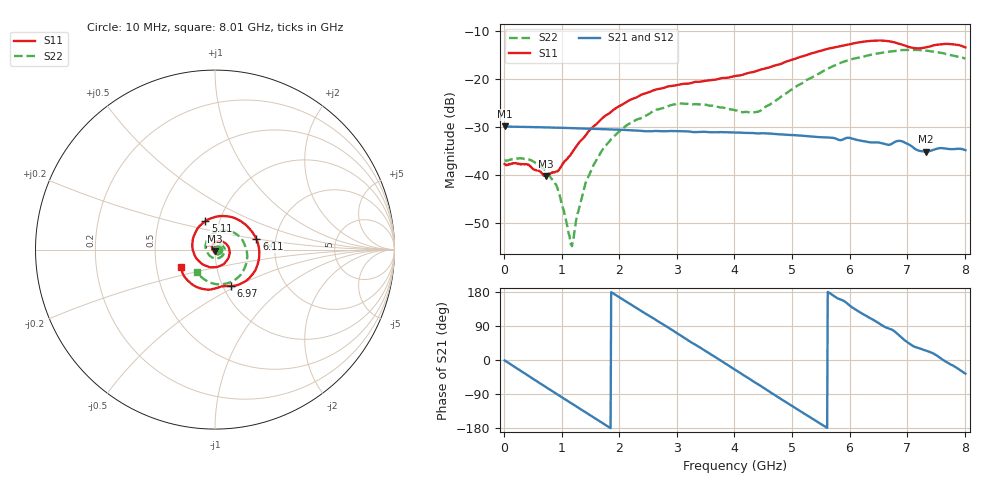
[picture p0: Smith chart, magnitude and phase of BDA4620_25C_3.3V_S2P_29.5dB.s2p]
!Agilent Technologies,E5071B,MY42404982,A.09.10
!Date: Wed May 06 08:55:15 2026
!Data & Calibration Information:
!Freq	S11:SOLT2(ON)	S21:SOLT2(ON)	S12:SOLT2(ON)	S22:SOLT2(ON)
# Hz S RI R 50
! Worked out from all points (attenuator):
!   801 points, 10 MHz to 8.01 GHz, reference 50 ohm
!   highest |S21| = -29.86 dB at 10 MHz (marker M1); lowest = -35.1 dB at 7.33 GHz (marker M2)
!   lowest |S11| = -40.2 dB at 720 MHz (marker M3), VSWR 1.02, Z = 49.8 - j0.961 ohm
!   |S11| at or under -10 dB: start of sweep to end of sweep
!   |S22| runs from -54.8 to -13.9 dB; largest |S21 - S12| = 0.0002
!   S11 on the Smith chart (normalised r, x): 10 MHz: 1.03, -0.00; 5.11 GHz: 0.86, +0.28; 6.11 GHz: 1.59, +0.19; 6.97 GHz: 1.09, -0.47; 8.01 GHz: 0.67, -0.14
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1e7  0.013 -0.000746  0.0321 -0.000672  0.0322 -0.000656  0.014 -0.000464
4.4e8  0.00856 -0.00926  0.023 -0.0218  0.023 -0.0218  0.0135 -0.00514
7.2e8  -0.00148 -0.00964  0.0103 -0.0296  0.0103 -0.0296  0.00851 -0.00729
9.3e8  -0.00959 -0.00526  -0.000679 -0.0311  -0.000697 -0.0311  0.00356 -0.00631
1.17e9  -0.0157 0.00595  -0.0128 -0.0281  -0.0129 -0.0281  -0.00158 -0.00111
1.2e9  -0.0161 0.00773  -0.0142 -0.0273  -0.0142 -0.0273  -0.00206 -8.8e-05
1.35e9  -0.0163 0.0168  -0.0204 -0.0228  -0.0204 -0.0228  -0.00355 0.00452
1.53e9  -0.0119 0.0288  -0.026 -0.0155  -0.0261 -0.0155  -0.00347 0.0112
1.77e9  0.00163 0.0418  -0.0297 -0.00404  -0.0298 -0.00404  0.000624 0.0204
2.15e9  0.0364 0.0462  -0.0258 0.0142  -0.0258 0.0143  0.0169 0.0292
2.68e9  0.0786 0.00593  -0.00575 0.0281  -0.00574 0.0282  0.0442 0.0196
3.08e9  0.0736 -0.0494  0.0128 0.0255  0.0129 0.0256  0.0551 -0.00704
4.01e9  -0.071 -0.0807  0.025 -0.012  0.0251 -0.0121  -0.0101 -0.0464
4.43e9  -0.1239 -0.00181  0.0111 -0.0248  0.0111 -0.0249  -0.0447 -0.0118
5.11e9  -0.054 0.1587  -0.0172 -0.0193  -0.0173 -0.0193  -0.0168 0.0848
5.35e9  0.0162 0.1852  -0.0228 -0.0107  -0.0228 -0.0107  0.0228 0.1016
6.11e9  0.2311 0.0574  -0.0158 0.0172  -0.0157 0.0174  0.16 0.04
6.68e9  0.1859 -0.1638  0.00248 0.0205  0.00254 0.0205  0.1698 -0.09
6.97e9  0.0898 -0.203  0.0137 0.0167  0.0138 0.0167  0.1305 -0.1525
7.33e9  0.0108 -0.2138  0.0159 0.00724  0.016 0.00728  0.0455 -0.1923
7.66e9  -0.1023 -0.2087  0.0189 -0.00115  0.0189 -0.00112  -0.035 -0.1803
8.01e9  -0.1898 -0.0987  0.0147 -0.0107  0.0147 -0.0106  -0.1015 -0.1275
